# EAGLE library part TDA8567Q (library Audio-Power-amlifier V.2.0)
The TDA8567Q is an integrated class-B output amplifier in a 23-lead Single-In-Line (SIL) plastic power package. It contains four amplifiers in BTL configuration, each with a gain of 26 dB. The output power is 4 ´ 25 W in a 4 W load.
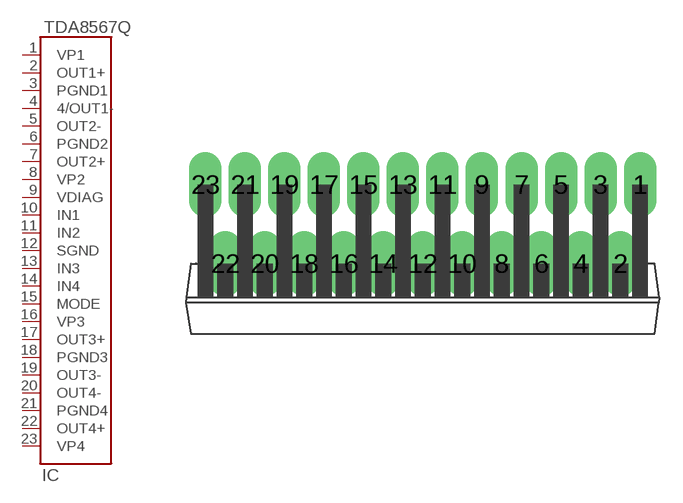
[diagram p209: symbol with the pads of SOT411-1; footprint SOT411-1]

Designator prefix IC

## TDA8567Q  [SOT411-1]
1  VP1  pwr
2  OUT1+  out
3  PGND1  pwr
4  4/OUT1-  out
5  OUT2-  out
6  PGND2  pwr
7  OUT2+  out
8  VP2  pwr
9  VDIAG  out
10  IN1  in
11  IN2  in
12  SGND  pwr
13  IN3  in
14  IN4  in
15  MODE  in
16  VP3  out
17  OUT3+  out
18  PGND3  pwr
19  OUT3-  out
20  OUT4-  out
21  PGND4  out
22  OUT4+  out
23  VP4  pwr

## Footprint SOT411-1 (pad centres in mm)
drill 1.4 long: 1 13.97,5.08; 2 12.7,0; 3 11.43,5.08; 4 10.16,0; 5 8.89,5.08; 6 7.62,0; 7 6.35,5.08; 8 5.08,0; 9 3.81,5.08; 10 2.54,0; 11 1.27,5.08; 12 0,0; 13 -1.27,5.08; 14 -2.54,0; 15 -3.81,5.08; 16 -5.08,0; 17 -6.35,5.08; 18 -7.62,0; 19 -8.89,5.08; 20 -10.16,0; 21 -11.43,5.08; 22 -12.7,0; 23 -13.97,5.08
